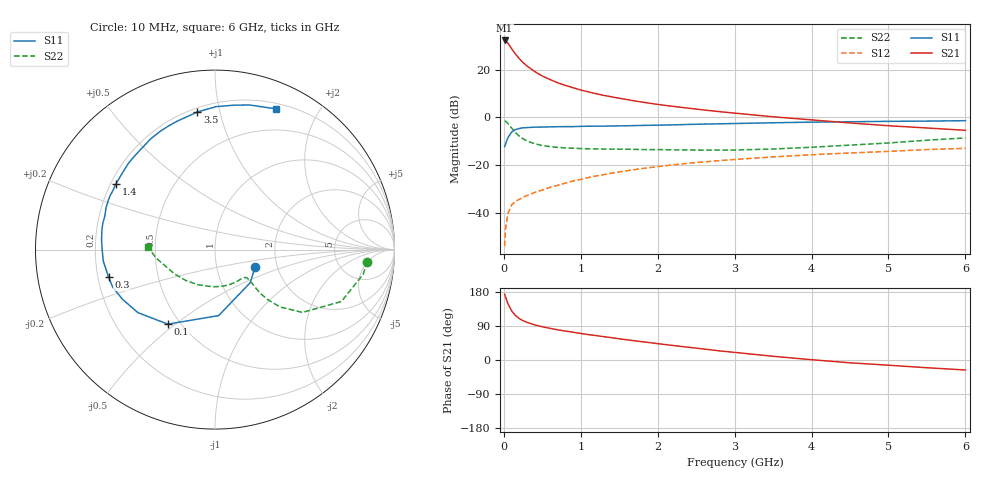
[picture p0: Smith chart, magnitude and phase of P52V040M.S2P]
! SIEMENS Small Signal Semiconductors
! BFP183
! Si NPN RF Bipolar Junction Transistor in SOT143
! VCE = 2 V  IC = 40 mA
! Common Emitter S-Parameters:  March  1996
# GHz  S  MA  R  50
!  f  S11  S21  S12  S22
! GHz  MAG  ANG  MAG  ANG  MAG  ANG  MAG  ANG
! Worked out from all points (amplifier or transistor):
!   36 points, 10 MHz to 6 GHz, reference 50 ohm
!   highest |S21| = 32.3 dB at 10 MHz (marker M1)
!   |S21| within 3 dB of that: start of sweep to 91.48 MHz
!   unconditionally stable (mu >= 1): start of sweep to 15.73 MHz; 333 MHz to end of sweep
!   at 250 MHz: K = 0.86, MSG = 28.2 dB, |S12| = -33.5 dB
!   at 1.4 GHz: K = 1.42, MAG = 12.2 dB, |S12| = -23.4 dB
!   at 6 GHz: K = 1.11, MAG = 1.8 dB, |S12| = -13.0 dB
!   S11 on the Smith chart (normalised r, x): 10 MHz: 1.54, -0.31; 100 MHz: 0.43, -0.47; 300 MHz: 0.24, -0.12; 1.4 GHz: 0.22, +0.29; 3.5 GHz: 0.22, +0.85; 6 GHz: 0.26, +1.49
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0.01  0.244 -23.0  41.1 173.6  0.002 72.9  0.8518 -4.5
0.02  0.2693 -43.5  40.66 167.5  0.0043 76.1  0.8367 -9.5
0.05  0.3681 -86.8  36.6 150.1  0.0094 68.8  0.7614 -22.3
0.1  0.4912 -122.3  27.76 130.0  0.0145 54.3  0.5998 -35.7
0.15  0.5549 -140.7  21.47 117.6  0.0175 48.6  0.4834 -41.4
0.2  0.5859 -152.0  17.14 109.4  0.0191 48.5  0.4056 -43.5
0.25  0.6069 -159.8  14.12 103.6  0.0212 49.0  0.3559 -43.9
0.3  0.6124 -165.6  12.03 99.5  0.023 50.1  0.321 -43.5
0.4  0.6255 -174.0  9.196 92.7  0.0267 53.1  0.2811 -42.4
0.5  0.6288 -179.9  7.376 87.7  0.03 54.2  0.2578 -41.7
0.6  0.6345 174.9  6.228 83.5  0.0344 57.0  0.244 -41.5
0.7  0.6393 170.3  5.329 79.7  0.0378 58.2  0.2354 -41.7
0.8  0.6421 166.8  4.703 76.3  0.042 58.9  0.2302 -42.4
1.1  0.6544 155.7  3.431 67.0  0.0551 59.7  0.2202 -46.4
1.4  0.6627 146.5  2.708 58.9  0.0678 58.9  0.2162 -52.2
1.8  0.6805 135.2  2.096 48.1  0.0849 56.0  0.2125 -61.7
2.2  0.6985 125.0  1.708 38.3  0.1014 52.5  0.2092 -72.6
2.8  0.735 111.0  1.325 24.1  0.1243 46.5  0.2074 -91.9
3.5  0.7728 97.3  1.032 9.8  0.1487 39.9  0.2179 -116.1
4.5  0.8123 82.2  0.766 -7.4  0.1798 30.0  0.2632 -149.1
5.5  0.838 71.6  0.601 -20.4  0.2119 21.2  0.3331 -172.2
6  0.8545 66.6  0.537 -26.4  0.225 16.1  0.3722 178.0
